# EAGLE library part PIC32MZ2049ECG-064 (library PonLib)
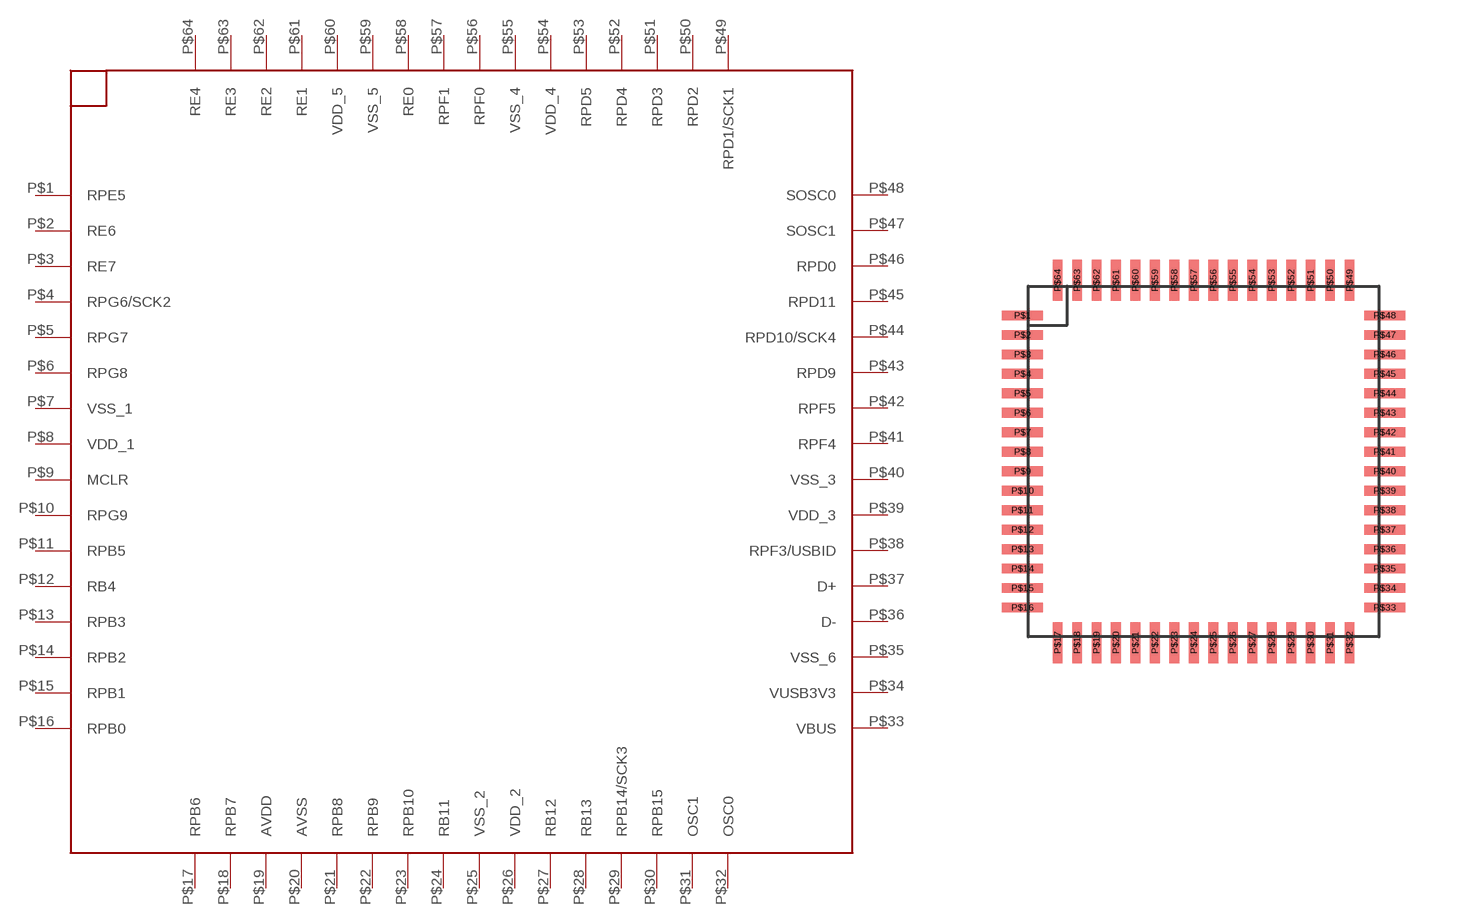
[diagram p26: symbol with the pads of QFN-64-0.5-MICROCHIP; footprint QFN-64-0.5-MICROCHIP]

Designator prefix -

## PIC32MZ2049ECG-064  [QFN-64-0.5-MICROCHIP]
P$1  RPE5
P$2  RE6
P$3  RE7
P$4  RPG6/SCK2
P$5  RPG7
P$6  RPG8
P$7  VSS_1
P$8  VDD_1
P$9  MCLR
P$10  RPG9
P$11  RPB5
P$12  RB4
P$13  RPB3
P$14  RPB2
P$15  RPB1
P$16  RPB0
P$17  RPB6
P$18  RPB7
P$19  AVDD
P$20  AVSS
P$21  RPB8
P$22  RPB9
P$23  RPB10
P$24  RB11
P$25  VSS_2
P$26  VDD_2
P$27  RB12
P$28  RB13
P$29  RPB14/SCK3
P$30  RPB15
P$31  OSC1
P$32  OSC0
P$33  VBUS
P$34  VUSB3V3
P$35  VSS_6
P$36  D-
P$37  D+
P$38  RPF3/USBID
P$39  VDD_3
P$40  VSS_3
P$41  RPF4
P$42  RPF5
P$43  RPD9
P$44  RPD10/SCK4
P$45  RPD11
P$46  RPD0
P$47  SOSC1
P$48  SOSC0
P$49  RPD1/SCK1
P$50  RPD2
P$51  RPD3
P$52  RPD4
P$53  RPD5
P$54  VDD_4
P$55  VSS_4
P$56  RPF0
P$57  RPF1
P$58  RE0
P$59  VSS_5
P$60  VDD_5
P$61  RE1
P$62  RE2
P$63  RE3
P$64  RE4

## Footprint QFN-64-0.5-MICROCHIP (pad centres in mm)
smd 1.05 x 0.25: P$1 -4.65,3.75; P$2 -4.65,3.25; P$3 -4.65,2.75; P$4 -4.65,2.25; P$5 -4.65,1.75; P$6 -4.65,1.25; P$7 -4.65,0.75; P$8 -4.65,0.25; P$9 -4.65,-0.25; P$10 -4.65,-0.75; P$11 -4.65,-1.25; P$12 -4.65,-1.75; P$13 -4.65,-2.25; P$14 -4.65,-2.75; P$15 -4.65,-3.25; P$16 -4.65,-3.75; P$33 4.65,-3.75; P$34 4.65,-3.25; P$35 4.65,-2.75; P$36 4.65,-2.25; P$37 4.65,-1.75; P$38 4.65,-1.25; P$39 4.65,-0.75; P$40 4.65,-0.25; P$41 4.65,0.25; P$42 4.65,0.75; P$43 4.65,1.25; P$44 4.65,1.75; P$45 4.65,2.25; P$46 4.65,2.75; P$47 4.65,3.25; P$48 4.65,3.75
smd 0.25 x 1.05: P$17 -3.75,-4.65; P$18 -3.25,-4.65; P$19 -2.75,-4.65; P$20 -2.25,-4.65; P$21 -1.75,-4.65; P$22 -1.25,-4.65; P$23 -0.75,-4.65; P$24 -0.25,-4.65; P$25 0.25,-4.65; P$26 0.75,-4.65; P$27 1.25,-4.65; P$28 1.75,-4.65; P$29 2.25,-4.65; P$30 2.75,-4.65; P$31 3.25,-4.65; P$32 3.75,-4.65; P$49 3.75,4.65; P$50 3.25,4.65; P$51 2.75,4.65; P$52 2.25,4.65; P$53 1.75,4.65; P$54 1.25,4.65; P$55 0.75,4.65; P$56 0.25,4.65; P$57 -0.25,4.65; P$58 -0.75,4.65; P$59 -1.25,4.65; P$60 -1.75,4.65; P$61 -2.25,4.65; P$62 -2.75,4.65; P$63 -3.25,4.65; P$64 -3.75,4.65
